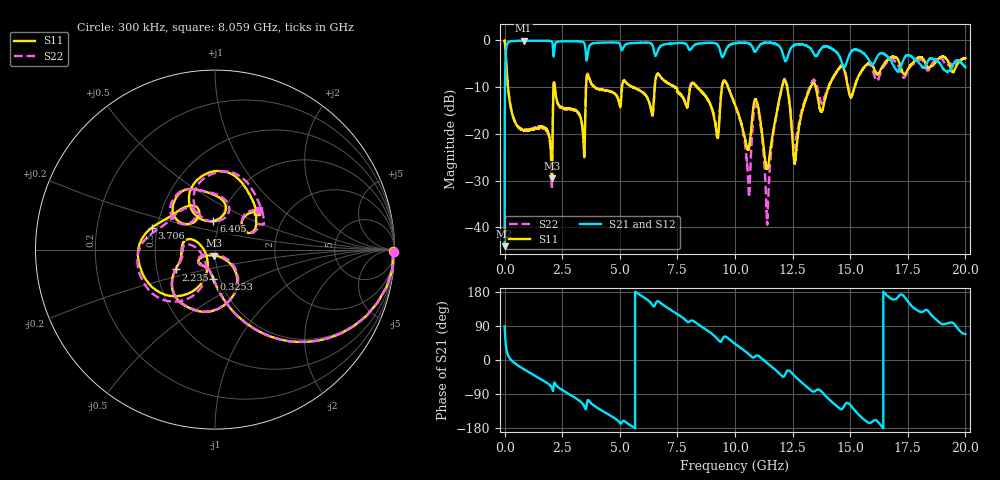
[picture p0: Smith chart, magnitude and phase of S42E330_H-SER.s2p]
!{S42E330}
!Johanson Technology Inc.
!www.johansontechnology.com
!Test Board Conditions:
!Substrate Type  RO4350B
!Substrate Thickness  50 mil
!Substrate Dk  3.66
!TL Type: GCPW
!TL Trace Width  60 mil
!TL Gap  10 mil
!Electrode orientation  Horizontal
!DUT TOPOLOGY	SERIES
!Mounting Pad LxW  14x55 mil
! Created Wed Nov 25 22:10:58 2020
# khz S ma R 50
! 2 Port Network Data from SP1.SP block
! freq  magS11  angS11  magS21  angS21  magS12  angS12  magS22  angS22
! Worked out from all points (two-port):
!   20001 points, 300 kHz to 20 GHz, reference 50 ohm
!   highest |S21| = -0.07 dB at 823.3 MHz (marker M1); lowest = -44.0 dB at 300 kHz (marker M2)
!   |S21| within 3 dB of the highest: 3.602 GHz to 6.519 GHz (2.917 GHz wide, 57.7 % of centre); 6.587 GHz to 9.399 GHz (2.812 GHz wide, 35.2 % of centre)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
!   lowest |S11| = -29.5 dB at 2.053 GHz (marker M3), VSWR 1.07, Z = 49.5 - j3.28 ohm
!   |S11| at or under -10 dB: 146.8 MHz to 2.12 GHz (1.973 GHz wide, 174 % of centre); 2.181 GHz to 3.536 GHz (1.355 GHz wide, 47.4 % of centre); 9.7 GHz to 12.04 GHz (2.338 GHz wide, 21.5 % of centre)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
!   |S22| runs from -39.5 to 0.0 dB; largest |S21 - S12| = 0.018
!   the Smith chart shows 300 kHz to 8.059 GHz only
!   S11 on the Smith chart (normalised r, x): 300 kHz: open; 325.3 MHz: 0.93, -0.32; 2.235 GHz: 0.63, -0.15; 3.706 GHz: 0.47, +0.13; 6.405 GHz: 0.93, +0.31; 8.059 GHz: 1.45, +0.66
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300  0.993 -0.5  0.006273 88.8  0.006361 89.0  0.9961 -0.6
108300  0.408 -69.9  0.9119 20.2  0.9116 20.1  0.4096 -69.9
325300  0.1651 -93.1  0.9836 -2.4  0.9842 -2.4  0.1666 -93.1
823300  0.1094 -114.7  0.9925 -23.9  0.9915 -23.9  0.1109 -114.8
2053300  0.0334 -97.0  0.9706 -73.7  0.9714 -73.7  0.0256 -95.9
2235300  0.246 -153.2  0.9537 -66.6  0.9548 -66.6  0.242 -153.6
3334300  0.1376 156.0  0.9757 -111.9  0.9754 -111.9  0.1358 169.0
3706300  0.3732 160.9  0.8883 -111.0  0.8897 -111.0  0.3706 167.2
4895300  0.2465 112.5  0.9488 -158.8  0.9487 -158.9  0.2476 117.2
6405300  0.1604 93.2  0.899 145.8  0.899 145.7  0.1587 85.9
6667300  0.4383 82.5  0.7928 154.9  0.791 154.9  0.4401 76.5
8059300  0.3154 40.9  0.7936 103.4  0.79 103.5  0.3314 41.3
1.00003e7  0.2057 -38.7  0.9337 42.7  0.9333 42.9  0.2049 -46.4
1.05903e7  0.06852 2.6  0.9293 15.7  0.9308 15.8  0.0255 -33.3
1.09703e7  0.2117 -26.3  0.8159 12.1  0.8173 12.3  0.1909 -35.2
1.13983e7  0.04228 2.2  0.947 -8.1  0.9459 -8.0  0.01086 -3.8
1.20943e7  0.356 9.1  0.6993 -44.1  0.7032 -44.1  0.3609 4.3
1.26013e7  0.04921 -9.4  0.8991 -42.9  0.9006 -43.1  0.07226 -20.9
1.33343e7  0.3349 -4.7  0.7849 -82.0  0.7866 -81.8  0.3558 -17.0
1.50973e7  0.2641 -64.5  0.7846 -125.7  0.7818 -125.8  0.265 -69.0
1.66673e7  0.6303 -107.4  0.6576 166.9  0.6423 166.9  0.6085 -112.9
2e7  0.6471 150.7  0.5163 68.5  0.5163 69.6  0.6358 152.9
